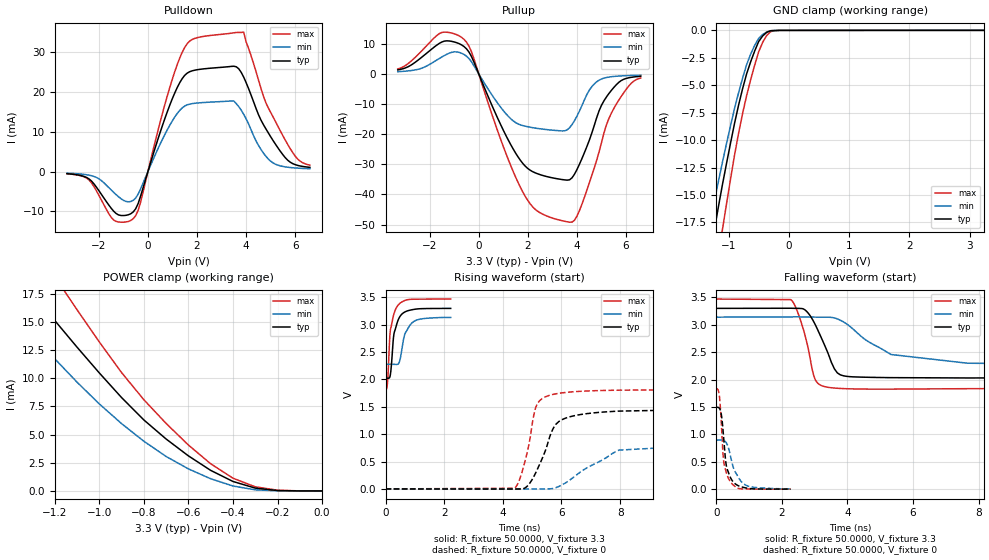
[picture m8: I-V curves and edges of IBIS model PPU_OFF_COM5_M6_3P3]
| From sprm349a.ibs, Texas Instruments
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|PPU_ON_IND5_M3_3P3BUFFER OPERATING AT 100UA IN SLOWEST MODE WITH INDTEMP AT
| PLUS OR MINUS 5PERCENT VDDS WITH PULLDOWN ON
|COM AND INDE ARE TWO DIFFERENT TEMP MODES.
|COM IS 25,0,105(NOM,STRONG,WEAK)
|IND IS 25,-40,125(NOM,STRONG,WEAK)
|   Model Cell PPU_OFF_COM5_M6_3P3
|PPU_OFF_COM5_M6_3P3
[Model]   PPU_OFF_COM5_M6_3P3
Model_type   I/O
Polarity   Non-Inverting
Enable   Active-Low
Vinl =  0.8V
Vinh =  2V
Cref =  15.0000pF
Rref =  100.0000M
Vref =  0V
Vmeas =  1.65
C_comp   1.471252p   1.43537p   1.511509p
[Model Spec]
Vinl   0.8V   0.8V   0.8V
Vinh   2V   2V   2V
[Temperature Range]   25   105   0
[Voltage Range]   3.3   3.14   3.47
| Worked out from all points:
|   slope of the pulldown table from 0 to 0.495 V, typ, clamps not added: 50.8 ohm
|   slope of the pullup table from 0 to 0.495 V, typ, clamps not added: 51.2 ohm
|   GND clamp passes 1 mA (typ) near -0.50 V on its own axis
|   POWER clamp passes 1 mA (typ) near -0.42 V on its own axis
|   rising waveform, R_fixture 50.0000, V_fixture 3.3: 20-80 % time 199ps typ, 272ps min, 167ps max; typ from 2.02 V to 3.3 V
|   rising waveform, R_fixture 50.0000, V_fixture 0: 20-80 % time 702ps typ, 1.67ns min, 424ps max; typ from 0 V to 1.49 V
|   falling waveform, R_fixture 50.0000, V_fixture 3.3: 20-80 % time 549ps typ, 1.47ns min, 404ps max; typ from 3.3 V to 2.04 V
|   falling waveform, R_fixture 50.0000, V_fixture 0: 20-80 % time 186ps typ, 319ps min, 150ps max; typ from 1.49 V to 0.002 V
[POWER_clamp]
|   voltage   I(typ)   I(min)   I(max)
-3.3V     77.67mA    59.59mA    94.92mA
-1.467V   22.04mA    17.66mA    27.25mA
-1.433V   21.11mA    16.9mA     26.17mA
-1.3V     17.58mA    13.9mA     22.02mA
-1.267V   16.76mA    13.17mA    21.02mA
-1.133V   13.55mA    10.34mA    17.06mA
-900mV    8.283mA    5.971mA    10.5mA
-800mV    6.297mA    4.41mA     8.092mA
-500mV    1.823mA    1.08mA     2.408mA
-400mV    839.2uA    436.8uA    1.129mA
-300mV    250.4uA    97.13uA    364.9uA
0V        112.2nA    125nA      532.4nA
[Pulldown]
|   voltage   I(typ)   I(min)   I(max)
-3.3V     -544.2uA   -400.3uA   -550.1uA
-2.4V     -1.845mA   -905.6uA   -2.119mA
-1.4V     -9.905mA   -5.191mA   -12.13mA
-600mV    -10.12mA   -7.213mA   -11.81mA
-300mV    -6.174mA   -4.366mA   -7.708mA
900mV     16.8mA     11.71mA    21.29mA
1.5V      24.11mA    16.42mA    31.12mA
3.5V      26.38mA    17.68mA    34.76mA
3.9V      23.67mA    14.35mA    34.94mA
4.9V      9.732mA    3.172mA    15.98mA
5.7V      2.814mA    1.083mA    6.746mA
6.6V      1.052mA    698.2uA    1.588mA
[Pullup]
|   voltage   I(typ)   I(min)   I(max)
-3.3V     1.324mA    742.3uA    1.642mA
-1.6V     10.17mA    5.149mA    13.4mA
-600mV    9.081mA    6.451mA    11.47mA
-300mV    5.824mA    4.053mA    7.407mA
1.1V      -20.32mA   -13.16mA   -26.27mA
1.9V      -30.67mA   -17.37mA   -40.73mA
2.5V      -33.44mA   -18.22mA   -46.11mA
3.7V      -35.15mA   -17.86mA   -49.23mA
4.2V      -28.16mA   -10.56mA   -43.32mA
5.2V      -7.672mA   -1.2mA     -16.95mA
6V        -1.511mA   -580.1uA   -5.196mA
6.6V      -790.2uA   -430.8uA   -1.375mA
[GND_clamp]
|   voltage   I(typ)   I(min)   I(max)
-3.3V     -92.33mA   -71.68mA   -112mA
-1.367V   -22.61mA   -19.11mA   -27.92mA
-1.3V     -20.3mA    -17.29mA   -25.34mA
-1.233V   -18.14mA   -15.51mA   -22.9mA
-1.1V     -14.04mA   -12mA      -18.13mA
-1.033V   -12.14mA   -10.32mA   -15.82mA
-900mV    -8.477mA   -7.121mA   -11.36mA
-700mV    -3.973mA   -3.129mA   -5.953mA
-500mV    -1.023mA   -735.9uA   -1.959mA
-366.7mV  -182.4uA   -147.3uA   -473.7uA
-166.7mV  -5.407uA   -5uA       -10.98uA
3.233V    80.37nA    1.447uA    401.5nA
[Ramp]
| variable   typ   min   max
dV/dt_f  0.7705802/0.5578131n  0.5283146/1.296293n   1.001384/0.409536n
dV/dt_r  0.8978509/0.7048709n  0.5372508/1.663926n   1.104406/0.4259007n
R_load = 50
[Rising Waveform]
R_fixture = 50.0000
V_fixture = 3.3
V_fixture_min = 3.14
V_fixture_max = 3.47
|   time   V(typ)   V(min)   V(max)
0s        2.024V     2.275V     1.813V
60ps      2.024V     2.278V     1.911V
135ps     2.033V     2.278V     2.707V
165ps     2.095V     2.278V     2.911V
270ps     2.777V     2.277V     3.172V
420ps     3.076V     2.28V      3.354V
495ps     3.156V     2.368V     3.395V
645ps     3.23V      2.812V     3.441V
900ps     3.274V     3.035V     3.465V
2.22ns    3.298V     3.133V     3.469V
[Rising Waveform]
R_fixture = 50.0000
V_fixture = 0
V_fixture_min = 0
V_fixture_max = 0
|   time   V(typ)   V(min)   V(max)
0s        52.07uV    27.79uV    83.03uV
4.395ns   -1.936mV   -1.255mV   12.58mV
4.68ns    4.164mV    -3.497mV   356.3mV
5.085ns   256mV      -375.5uV   1.419V
5.235ns   426.8mV    -109.7uV   1.6V
5.91ns    1.231V     45.19mV    1.747V
7.215ns   1.396V     479.5mV    1.796V
7.965ns   1.422V     709.4mV    1.805V
16.93ns   1.474V     866.5mV    1.821V
115.5ns   1.487V     887.9mV    1.833V
[Falling Waveform]
R_fixture = 50.0000
V_fixture = 3.3
V_fixture_min = 3.14
V_fixture_max = 3.47
|   time   V(typ)   V(min)   V(max)
0s        3.3V       3.14V      3.47V
2.265ns   3.302V     3.144V     3.46V
2.625ns   3.295V     3.143V     2.972V
2.955ns   3.073V     3.14V      2.107V
3.045ns   2.967V     3.14V      1.969V
3.6ns     2.197V     3.126V     1.846V
3.87ns    2.07V      3.056V     1.836V
5.325ns   2.036V     2.458V     1.826V
7.665ns   2.03V      2.299V     1.834V
61.52ns   2.039V     2.268V     1.82V
[Falling Waveform]
R_fixture = 50.0000
V_fixture = 0
V_fixture_min = 0
V_fixture_max = 0
|   time   V(typ)   V(min)   V(max)
0s        1.493V     895.8mV    1.834V
90ps      1.476V     897.3mV    1.701V
165ps     1.295V     897.5mV    1.02V
195ps     1.12V      894.3mV    688mV
225ps     902mV      887.8mV    488.8mV
300ps     435.1mV    847.2mV    306.8mV
435ps     203.5mV    587mV      128.5mV
570ps     99.25mV    317.9mV    47.71mV
885ps     24.66mV    76.41mV    3.809mV
2.265ns   1.516mV    6.443mV    475.7uV
